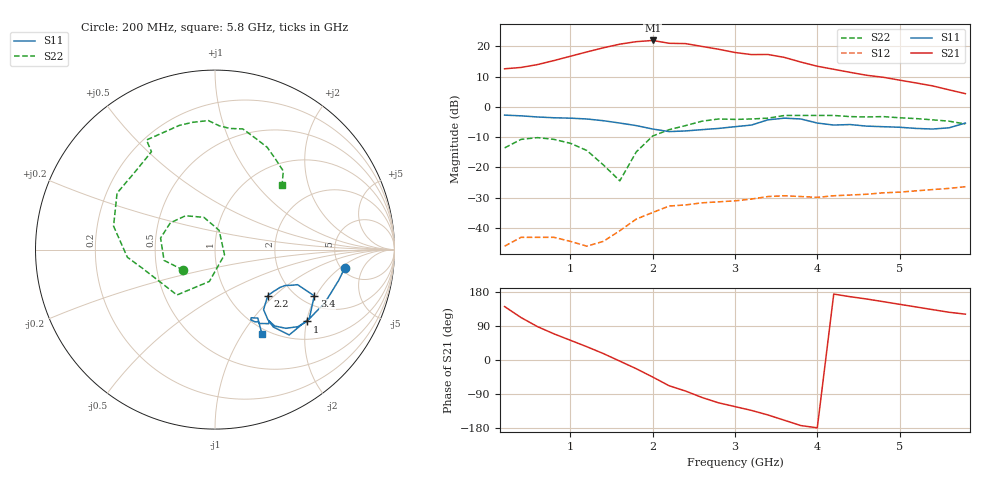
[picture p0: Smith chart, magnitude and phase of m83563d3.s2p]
!	MGA-83563 S PARAMETERS
!	Vd = 3 V L=2.2 nH  LAST UPDATED 10-15-97
# ghz	s ma r	50
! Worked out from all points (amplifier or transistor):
!   29 points, 200 MHz to 5.8 GHz, reference 50 ohm
!   highest |S21| = 21.9 dB at 2 GHz (marker M1)
!   |S21| within 3 dB of that: 1.316 GHz to 2.817 GHz (1.502 GHz wide, 72.7 % of centre)
!   unconditionally stable (mu >= 1): start of sweep to end of sweep
!   at 1 GHz: K = 6.45, MAG = 19.5 dB, |S12| = -44.4 dB
!   at 3 GHz: K = 1.49, MAG = 20.4 dB, |S12| = -31.1 dB
!   at 5.8 GHz: K = 3.55, MAG = 6.9 dB, |S12| = -26.4 dB
!   S11 on the Smith chart (normalised r, x): 200 MHz: 5.36, -2.33; 1 GHz: 1.45, -2.01; 2.2 GHz: 1.50, -0.91; 3.4 GHz: 2.36, -1.94; 5.8 GHz: 0.92, -1.23
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0.2  0.73 -8.0  4.25 141.0  0.005 59.0  0.21 -147.0
0.4  0.71 -14.0  4.47 112.0  0.007 41.0  0.29 -168.0
0.6  0.68 -26.0  4.99 88.0  0.007 30.0  0.31 168.0
0.8  0.66 -32.0  5.81 69.0  0.007 27.0  0.29 149.0
1  0.65 -38.0  6.85 52.0  0.006 35.0  0.25 131.0
1.2  0.63 -43.0  8.07 35.0  0.005 51.0  0.19 109.0
1.4  0.59 -48.0  9.44 17.0  0.006 78.0  0.11 78.0
1.6  0.54 -52.0  10.84 -3.0  0.009 91.0  0.06 -28.0
1.8  0.49 -53.0  11.92 -23.0  0.014 90.0  0.18 -100.0
2  0.43 -51.0  12.48 -45.0  0.018 85.0  0.33 -130.0
2.2  0.39 -41.0  11.21 -68.0  0.023 73.0  0.42 -166.0
2.4  0.4 -36.0  11.07 -82.0  0.024 68.0  0.49 -175.0
2.6  0.42 -30.0  9.94 -99.0  0.026 61.0  0.58 167.0
2.8  0.44 -27.0  8.93 -113.0  0.027 56.0  0.63 150.0
3  0.47 -25.0  7.9 -123.0  0.028 52.0  0.62 138.0
3.4  0.61 -25.0  7.32 -145.0  0.033 46.0  0.65 123.0
3.6  0.65 -36.0  6.55 -159.0  0.034 41.0  0.72 122.0
3.8  0.63 -49.0  5.49 -173.0  0.033 34.0  0.72 106.0
4  0.54 -53.0  4.68 -179.0  0.032 35.0  0.72 100.0
4.4  0.51 -54.0  3.71 167.0  0.035 34.0  0.69 88.0
5  0.46 -61.0  2.76 147.0  0.039 28.0  0.66 70.0
5.8  0.54 -61.0  1.65 121.0  0.048 16.0  0.52 44.0
